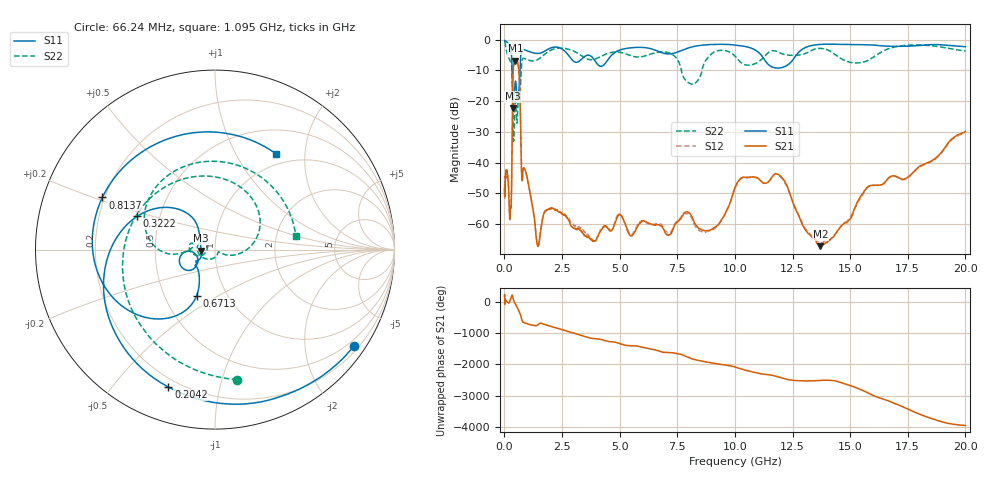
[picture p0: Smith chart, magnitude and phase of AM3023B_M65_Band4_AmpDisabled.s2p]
!Agilent Technologies,E8364B,MY43040894,A.07.50.67
!Agilent E8364B: A.07.50.67
!Date: Tuesday, October 27, 2020 10:49:13
!Correction: S11(Full 2 Port(1,2))
!S21(Full 2 Port(1,2))
!S12(Full 2 Port(1,2))
!S22(Full 2 Port(1,2))
!S2P File: Measurements: S11, S21, S12, S22:Log Frequency Sweep
# Hz S  dB  R 50
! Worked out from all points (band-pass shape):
!   3201 points, 10 MHz to 20 GHz, reference 50 ohm
!   highest |S21| = -6.82 dB at 474.6 MHz (marker M1); lowest = -67.2 dB at 13.71 GHz (marker M2)
!   |S21| within 3 dB of the highest: 385.2 MHz to 624.5 MHz (239.3 MHz wide, 47.4 % of centre)
!   lowest |S11| = -22.3 dB at 374.2 MHz (marker M3), VSWR 1.17, Z = 42.9 - j0.48 ohm
!   |S11| at or under -10 dB: 337.1 MHz to 677 MHz (339.9 MHz wide, 67 % of centre)
!   |S22| runs from -33.1 to -0.7 dB; largest |S21 - S12| = 0.0074
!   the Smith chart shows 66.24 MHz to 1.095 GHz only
!   S11 on the Smith chart (normalised r, x): 66.24 MHz: 0.33, -3.15; 204.2 MHz: 0.16, -0.70; 322.2 MHz: 0.37, +0.18; 671.3 MHz: 0.72, -0.40; 813.7 MHz: 0.19, +0.21; 1.095 GHz: 0.83, +1.48
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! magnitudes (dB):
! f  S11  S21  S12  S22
! 10 MHz  -0.3  -48.8  -44.6  -0.7
! 35.55 MHz  -0.4  -46.6  -46.5  -1.4
! 66.24 MHz  -0.5  -43.3  -44.1  -2.7
! 126.1 MHz  -1.0  -43.4  -43.3  -4.6
! 204.2 MHz  -1.8  -52.8  -51.7  -6.2
! 241.7 MHz  -2.5  -57.8  -58.3  -6.7
! 322.2 MHz  -6.5  -42.7  -42.5  -9.0
! 374.2 MHz  -22.3  -11.7  -11.8  -26.4
! 447.2 MHz  -16.1  -6.9  -7.0  -23.1
! 474.6 MHz  -13.7  -6.8  -6.9  -20.2
! 671.3 MHz  -11.2  -16.7  -16.7  -18.0
! 748.8 MHz  -3.5  -43.6  -43.7  -7.9
! 813.7 MHz  -3.2  -42.2  -42.3  -6.2
! 1.095 GHz  -4.0  -48.9  -48.9  -6.8
! 1.432 GHz  -4.5  -66.6  -66.2  -6.6
! 1.59 GHz  -4.3  -61.4  -60.9  -5.8
! 5.639 GHz  -2.6  -62.8  -62.4  -5.6
! 8.11 GHz  -2.4  -57.2  -57.8  -14.5
! 8.897 GHz  -1.6  -62.1  -62.3  -5.3
! 11.75 GHz  -9.2  -43.7  -43.8  -3.7
! 13.71 GHz  -1.6  -67.2  -66.0  -2.9
! 20 GHz  -2.3  -30.0  -30.3  -3.7
